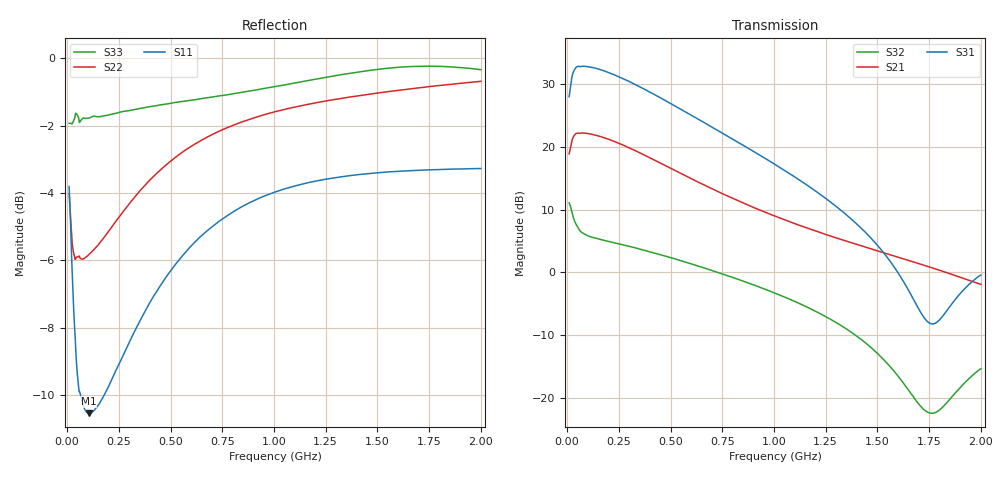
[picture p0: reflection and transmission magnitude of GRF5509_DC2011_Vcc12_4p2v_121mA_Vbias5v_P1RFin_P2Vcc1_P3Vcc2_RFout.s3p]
!Keysight Technologies,N5244B,MY57181157,A.18.40.03
!Date: Wednesday, April 29, 2026 14:27:19
!Correction: S11(C  3-Port  )
!S12(C  3-Port  )
!S13(C  3-Port  )
!S21(C  3-Port  )
!S22(C  3-Port  )
!S23(C  3-Port  )
!S31(C  3-Port  )
!S32(C  3-Port  )
!S33(C  3-Port  )
!S3P File: Measurements: <S11,S12,S13>,
!<S21,S22,S23>,
!<S31,S32,S33>:
# Hz S  dB  R 50
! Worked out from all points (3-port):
!   1991 points, 10 MHz to 2 GHz, reference 50 ohm
!   strongest paths, dB at 10 MHz, 507 MHz, 1.005 GHz, 1.503 GHz, 2 GHz:
!     S31: 28.0, 26.8, 17.2, 4.2, -0.4
!     S21: 18.9, 16.5, 9.0, 3.4, -1.9
!     S32: 11.1, 2.3, -3.3, -13.0, -15.4
!   lowest |S11| = -10.5 dB at 105 MHz (marker M1), VSWR 1.84, Z = 30.6 - j14.6 ohm
!   |S11| at or under -10 dB: 65.12 MHz to 179.4 MHz (114.3 MHz wide, 93.5 % of centre)
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1e7  -3.81 -53.8  -22.23 -34.2  -64.17 -154.3
     18.91 -137.0  -4.03 -78.7  -32.11 -87.0
     28.02 78.0  11.10 -173.7  -1.93 -113.2
3e7  -7.16 -91.1  -26.66 -42.8  -65.41 158.5
     21.58 -161.7  -5.73 -122.7  -43.19 144.2
     31.93 32.5  8.81 162.0  -1.87 -148.1
4.4e7  -8.89 -108.6  -28.71 -42.4  -64.13 -63.4
       22.16 -172.8  -5.92 -136.8  -42.71 -38.0
       32.71 16.2  7.67 158.3  -1.64 -158.4
1.05e8  -10.55 -132.8  -32.35 -31.1  -72.65 27.5
        22.13 163.4  -5.83 -156.9  -50.83 32.1
        32.79 -16.8  5.77 154.2  -1.78 -169.6
1.73e8  -10.08 -138.3  -33.35 -25.8  -71.26 89.3
        21.55 146.0  -5.37 -161.2  -45.32 43.8
        32.21 -39.1  5.16 147.4  -1.72 -172.2
2.53e8  -9.06 -140.0  -33.88 -24.6  -67.50 60.5
        20.56 129.2  -4.70 -163.5  -42.50 42.9
        31.17 -60.2  4.54 138.2  -1.61 -173.0
4.76e8  -6.52 -144.9  -35.05 -26.5  -61.21 86.0
        17.01 94.8  -3.18 -169.8  -39.77 32.4
        27.39 -106.4  2.59 113.3  -1.36 -173.2
6.69e8  -5.16 -150.5  -36.02 -28.5  -58.28 82.9
        13.83 75.1  -2.37 -175.0  -39.38 27.6
        23.77 -136.3  0.64 94.3  -1.18 -173.0
1.005e9  -3.97 -159.6  -37.41 -29.3  -54.91 85.3
         8.97 53.2  -1.59 177.9  -40.08 29.8
         17.22 -176.8  -3.30 65.9  -0.84 -173.3
2e9  -3.27 -178.5  -40.40 -42.6  -48.20 90.8
     -1.91 10.5  -0.68 156.3  -34.91 71.3
     -0.43 -126.4  -15.39 122.6  -0.34 172.2
